// ===========================================================================
// UDT741

// Datum	  Name	Aktion
// ---------------------------------------------------------------------------
// 30.10.97 Vetter	Neu

TYPE "XC_ASTA_UDT"

STRUCT
	bSrcPCU		: BYTE;		//Quell-PCU-Nummer
	bDestPCU		: BYTE;		//Ziel-PCU-Nummer
	bSrcASTA		: BYTE;		//Quell-ASTA
	bDestSEQ		: BYTE;		//Ziel-Teilanlage
	bYear			: BYTE;
	bRecipeType	: BYTE;
	iRecipe		: INT;
	iOrder		: INT;
	iBatch		: INT;
END_STRUCT

END_TYPE
